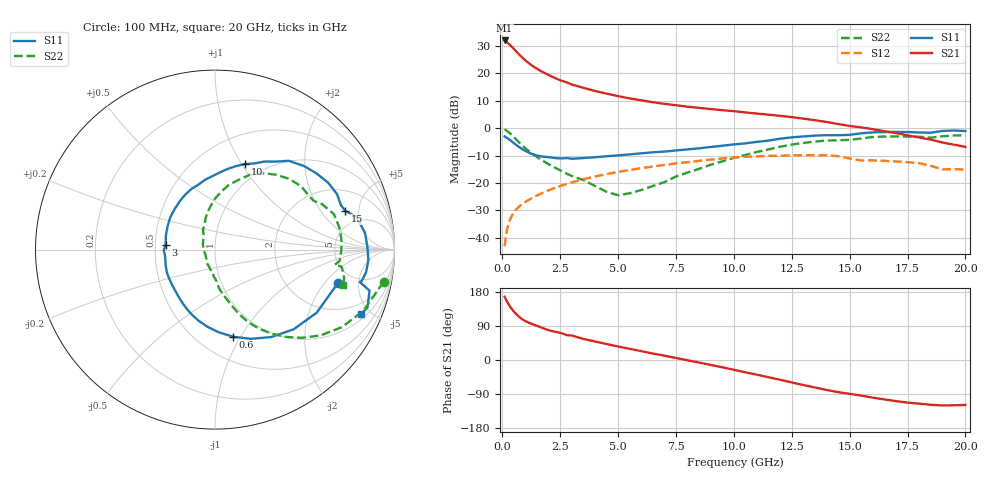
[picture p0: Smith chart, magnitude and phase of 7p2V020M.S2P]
! Infineon Technologies  Discrete & RF Semiconductors
! bfp620
! VCE =  2.0 V,  IC =  20 mA
! Common Emitter S-Parameters:  Sep 2002
# GHz  S  MA  R  50
!  f  S11  S21  S12  S22
! GHz  MAG  ANG  MAG  ANG  MAG  ANG  MAG  ANG
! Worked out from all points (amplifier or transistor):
!   59 points, 100 MHz to 20 GHz, reference 50 ohm
!   highest |S21| = 32.1 dB at 100 MHz (marker M1)
!   |S21| within 3 dB of that: start of sweep to 488.7 MHz
!   unconditionally stable (mu >= 1): 3.312 GHz to 9.969 GHz; 17.16 GHz to end of sweep
!   at 1 GHz: K = 0.69, MSG = 25.8 dB, |S12| = -26.9 dB
!   at 5.5 GHz: K = 1.04, MAG = 11.8 dB, |S12| = -15.3 dB
!   at 20 GHz: K = 1.29, MAG = 0.9 dB, |S12| = -15.1 dB
!   S11 on the Smith chart (normalised r, x): 100 MHz: 3.67, -2.78; 600 MHz: 0.72, -0.93; 3 GHz: 0.57, +0.03; 10 GHz: 0.81, +1.04; 15 GHz: 3.50, +3.53; 20 GHz: 1.26, -4.35
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0.1  0.7089 -15.4  40.1 167.0  0.007 71.4  0.9563 -10.8
0.2  0.6668 -31.8  37.1 154.4  0.014 71.1  0.8951 -22.3
0.3  0.6239 -45.4  34.09 144.1  0.0198 68.2  0.8289 -31.4
0.4  0.5791 -57.3  31.03 135.5  0.0247 65.3  0.759 -39.0
0.5  0.5355 -68.2  28.07 127.9  0.029 62.8  0.6894 -45.5
0.6  0.4959 -78.2  25.32 121.3  0.0327 60.7  0.6238 -51.2
0.7  0.4613 -87.4  22.87 115.5  0.0362 59.1  0.5645 -56.0
0.9  0.4064 -103.1  18.89 106.2  0.0423 57.0  0.4671 -63.6
1.1  0.3657 -115.5  15.98 99.6  0.048 55.9  0.3948 -68.7
1.3  0.3361 -125.9  13.83 94.7  0.0535 55.0  0.3406 -72.3
2  0.2953 -155.9  9.373 78.7  0.0733 52.0  0.2203 -83.5
2.8  0.2855 -179.5  6.845 65.3  0.0965 47.1  0.1469 -93.6
3  0.2765 174.7  6.287 64.8  0.1022 45.7  0.134 -93.4
3.5  0.2851 163.7  5.473 55.6  0.1169 41.8  0.1129 -103.3
5  0.3186 134.8  3.856 35.6  0.1591 29.0  0.0597 -154.8
7  0.374 104.1  2.787 11.5  0.2134 10.9  0.1033 128.1
10  0.5052 70.7  2.048 -25.8  0.2921 -21.1  0.2863 89.6
10.5  0.5291 65.2  1.944 -32.6  0.2998 -27.6  0.3248 83.8
13.5  0.7322 30.7  1.4 -72.5  0.3206 -63.1  0.5702 43.8
15  0.7562 16.6  1.101 -89.3  0.2803 -84.0  0.6127 26.4
17  0.8566 -3.9  0.814 -108.5  0.247 -94.7  0.7068 4.2
20  0.8889 -24.0  0.456 -118.6  0.1753 -105.0  0.741 -15.5
